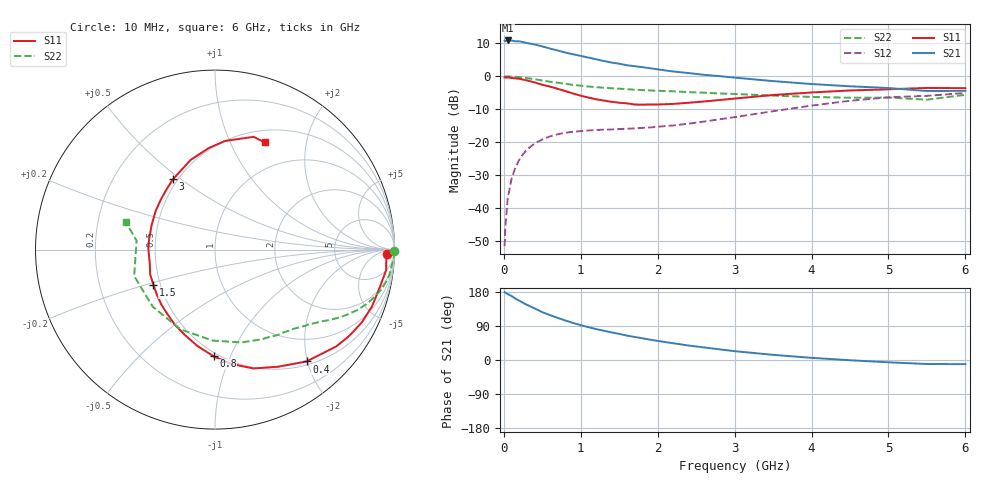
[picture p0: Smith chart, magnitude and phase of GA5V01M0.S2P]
! Infineon Technologies  Discrete & RF Semiconductors
! BF775
! Si NPN RF Bipolar Junction Transistor in SOT23
! VCE = 5 V  IC = 1 mA
! Common Emitter S-Parameters:  May  1996
# GHz  S  MA  R  50
!  f  S11  S21  S12  S22
! GHz  MAG  ANG  MAG  ANG  MAG  ANG  MAG  ANG
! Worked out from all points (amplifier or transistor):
!   36 points, 10 MHz to 6 GHz, reference 50 ohm
!   highest |S21| = 10.9 dB at 50 MHz (marker M1)
!   |S21| within 3 dB of that: start of sweep to 691.3 MHz
!   unconditionally stable (mu >= 1): 1.452 GHz to 3.779 GHz; 5.181 GHz to end of sweep
!   at 250 MHz: K = 0.20, MSG = 17.1 dB, |S12| = -23.7 dB
!   at 1.4 GHz: K = 0.98, MSG = 10.2 dB, |S12| = -16.2 dB
!   at 6 GHz: K = 1.02, MAG = -0.4 dB, |S12| = -5.1 dB
!   S11 on the Smith chart (normalised r, x): 10 MHz: 36, -22; 400 MHz: 0.56, -1.98; 800 MHz: 0.47, -0.87; 1.5 GHz: 0.46, -0.21; 3 GHz: 0.47, +0.47; 6 GHz: 0.64, +1.36
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0.01  0.9609 -1.4  3.469 179.2  0.0026 88.4  0.9999 -0.5
0.02  0.9552 -2.5  3.408 177.5  0.0052 84.4  0.997 -1.1
0.05  0.9605 -6.8  3.501 174.3  0.0138 85.3  0.9963 -2.8
0.1  0.9408 -13.3  3.484 168.7  0.0275 82.5  0.9872 -5.5
0.15  0.9301 -19.9  3.403 162.0  0.0409 77.5  0.9815 -8.3
0.2  0.9131 -26.4  3.395 156.6  0.0536 74.0  0.9694 -10.7
0.25  0.8884 -32.9  3.312 151.0  0.0651 69.6  0.9535 -13.3
0.4  0.8051 -50.7  3.048 136.1  0.0948 60.0  0.9006 -19.5
0.5  0.7412 -61.7  2.837 126.2  0.1095 54.3  0.8602 -23.1
0.6  0.696 -72.1  2.637 118.5  0.1216 49.6  0.8256 -25.8
0.8  0.5944 -90.8  2.288 104.1  0.1381 42.6  0.7657 -30.3
0.9  0.5461 -100.3  2.158 97.7  0.1432 40.3  0.7398 -32.2
1.1  0.4741 -118.3  1.922 86.7  0.1497 36.9  0.6978 -35.7
1.5  0.3953 -150.2  1.55 68.9  0.1571 34.8  0.6457 -41.6
1.9  0.3721 177.6  1.323 53.7  0.1661 37.9  0.6081 -48.3
2.2  0.3789 158.7  1.181 44.2  0.1782 40.5  0.5898 -53.9
3  0.4572 120.7  0.952 23.3  0.2386 45.6  0.5376 -74.2
3.5  0.5183 105.1  0.843 13.6  0.2937 44.3  0.507 -91.5
4.5  0.6075 84.8  0.703 -0.6  0.4233 33.3  0.4706 -137.5
5  0.6329 77.3  0.662 -6.1  0.4783 25.2  0.4738 -161.9
5.5  0.6641 71.1  0.596 -10.6  0.5032 15.8  0.4397 173.5
6  0.6584 65.2  0.599 -10.9  0.5564 10.9  0.5208 162.8
